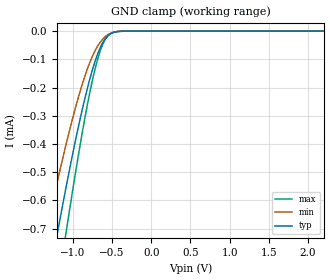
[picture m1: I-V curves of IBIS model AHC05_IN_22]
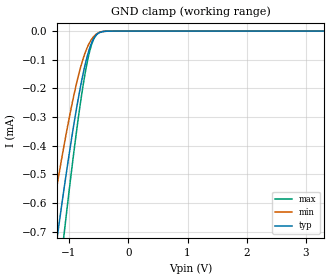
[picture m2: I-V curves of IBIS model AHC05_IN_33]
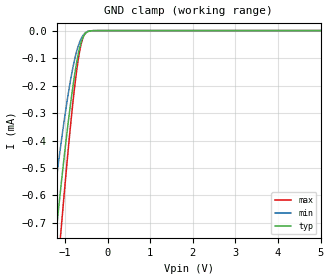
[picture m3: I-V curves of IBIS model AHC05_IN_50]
| TEXAS INSTRUMENTS INCORPORATED
| Standard Linear and Logic Group
| IBIS Model of SN74AHC05
| HEX INVERTERS WITH OPEN-DRAIN OUTPUTS
| This file contains package information for the following:
|  TSSOP 14-pin (PW) package as [Component] AHC05_PD_PW
|  PDIP 14-pin (N) package as [Component] AHC05_PD_N
|  SSOP 14-pin (DB) package as [Component] AHC05_PD_DB
|  SOIC 14-pin (D) package as [Component] AHC05_PD_D
|  TVSOP 14-pin (DGV) package as [Component] AHC05_PD_DGV
| This device can be powered at the following Vccs:
|  2.2 volt Vcc
|  3.3 volt Vcc
|  5 volt Vcc
| This file provides unique models under the [Model Selector] for each Vcc.
| For operation at a specific Vcc, select the appropriate model after each
| [Model Selector] keyword.
[IBIS Ver]   3.2
[Comment char]  |_char
[File Name]   sn74ahc05.ibs
[File Rev]   1.1 | i_die
[Date]   August 22, 2002
[Source]   Data created from TI-SPICE simulations at TI-SLL.
[Notes]   The following is an IBIS list for the AHC05_PD.
   Please contact sllibis@ti.com with questions and
   comments concerning SLL IBIS models.
[Disclaimer] Property of Texas Instruments Incorporated.  Unauthorized
   reproduction and/or distribution is strictly prohibited.
   This product is protected under copyright law.
   Created  2002, (C) Copyright  2002, Texas Instruments
   Incorporated, All Rights Reserved
   UNLESS THERE IS A SIGNED, WRITTEN AGREEMENT TO THE
   CONTRARY, TEXAS INSTRUMENTS (TI) IS PROVIDING THE IBIS
   MODELS  AND WITHOUT ANY WARRANTY, EXPRESSED OR
   IMPLIED.  TI assumes no liability for:
   1) the accuracy of the IBIS models provided to your
   company;
   2) the proper functioning of these IBIS Models in your
   design or for any resulting applications; or
   3) infringement of patents, copyrights or intellectual
   property rights resulting from your use of these IBIS
   models.
   TI provides IBIS Models as a service to our customers.
   You and your company shall not distribute, sell or give
   these models to anyone else without prior written
   permission from TI.
   TI reserves the right to make changes to our products or
   to discontinue any semiconductor product or service
   without notice, and advises our customers to obtain the
   latest version of relevant information to verify, before
   placing orders, that the information being relied on is
   current.
   Please be aware that your receipt and use of the IBIS
   information provided shall serve as acceptance of these
   terms and conditions.  If you do not accept these terms,
   you should return or destroy the IBIS models and any
   other accompanying information immediately.
| Component AHC05_PD_PW 14-pin TSSOP
[Component]   AHC05_PW
[Manufacturer]   Texas Instruments, Inc.
[Package]
|   typ   min   max
R_pkg   3.200e-02   2.900e-02   3.500e-02
L_pkg   2.378e-09   2.170e-09   2.680e-09
C_pkg   3.140e-13   2.700e-13   3.350e-13
[Pin]   signal_name   model_name   R_pin   L_pin   C_pin
1   1A   AHC05_IN   3.300e-02   2.618e-09   3.300e-13
2   1Y   AHC05_OUT   3.100e-02   2.313e-09   3.170e-13
3   2A   AHC05_IN   3.000e-02   2.310e-09   3.140e-13
4   2Y   AHC05_OUT   3.100e-02   2.173e-09   2.720e-13
5   3A   AHC05_IN   3.000e-02   2.204e-09   3.090e-13
6   3Y   AHC05_OUT   3.200e-02   2.315e-09   3.170e-13
7   GND   GND   3.500e-02   2.680e-09   3.350e-13
8   4Y   AHC05_OUT   3.300e-02   2.640e-09   3.330e-13
9   4A   AHC05_IN   3.400e-02   2.347e-09   3.190e-13
10   5Y   AHC05_OUT   2.900e-02   2.277e-09   3.130e-13
11   5A   AHC05_IN   3.100e-02   2.170e-09   2.700e-13
12   6Y   AHC05_OUT   3.100e-02   2.244e-09   3.110e-13
13   6A   AHC05_IN   3.300e-02   2.343e-09   3.210e-13
14   VCC   POWER   3.500e-02   2.657e-09   3.320e-13
| Component AHC05_PD_N 14-pin PDIP
[Component]   AHC05_N
[Manufacturer]   Texas Instruments, Inc.
[Package]
|   typ   min   max
R_pkg   4.500e-02   3.700e-02   6.300e-02
L_pkg   5.407e-09   3.922e-09   6.942e-09
C_pkg   3.890e-13   2.050e-13   6.040e-13
[Pin]   signal_name   model_name   R_pin   L_pin   C_pin
1   1A   AHC05_IN   6.300e-02   6.942e-09   6.040e-13
2   1Y   AHC05_OUT   3.700e-02   6.200e-09   4.060e-13
3   2A   AHC05_IN   4.200e-02   4.389e-09   3.220e-13
4   2Y   AHC05_OUT   3.800e-02   3.922e-09   2.050e-13
5   3A   AHC05_IN   3.900e-02   4.301e-09   2.980e-13
6   3Y   AHC05_OUT   3.800e-02   5.329e-09   3.560e-13
7   GND   GND   5.300e-02   6.510e-09   5.440e-13
8   4Y   AHC05_OUT   5.300e-02   6.437e-09   5.390e-13
9   4A   AHC05_IN   3.900e-02   5.352e-09   3.470e-13
10   5Y   AHC05_OUT   4.200e-02   4.473e-09   2.970e-13
11   5A   AHC05_IN   4.400e-02   4.326e-09   2.250e-13
12   6Y   AHC05_OUT   4.200e-02   4.295e-09   2.800e-13
13   6A   AHC05_IN   4.200e-02   6.318e-09   4.180e-13
14   VCC   POWER   6.100e-02   6.900e-09   6.030e-13
| Component AHC05_PD_DB 14-pin SSOP
[Component]   AHC05_DB
[Manufacturer]   Texas Instruments, Inc.
[Package]
|   typ   min   max
R_pkg   4.400e-02   4.100e-02   4.600e-02
L_pkg   3.551e-09   3.258e-09   3.927e-09
C_pkg   4.020e-13   3.600e-13   4.210e-13
[Pin]   signal_name   model_name   R_pin   L_pin   C_pin
1   1A   AHC05_IN   4.600e-02   3.927e-09   4.080e-13
2   1Y   AHC05_OUT   4.400e-02   3.587e-09   4.210e-13
3   2A   AHC05_IN   4.100e-02   3.289e-09   3.980e-13
4   2Y   AHC05_OUT   4.200e-02   3.258e-09   3.600e-13
5   3A   AHC05_IN   4.100e-02   3.286e-09   4.030e-13
6   3Y   AHC05_OUT   4.400e-02   3.586e-09   4.210e-13
7   GND   GND   4.600e-02   3.927e-09   4.080e-13
8   4Y   AHC05_OUT   4.600e-02   3.927e-09   4.080e-13
9   4A   AHC05_IN   4.400e-02   3.586e-09   4.210e-13
10   5Y   AHC05_OUT   4.100e-02   3.286e-09   4.030e-13
11   5A   AHC05_IN   4.300e-02   3.258e-09   3.600e-13
12   6Y   AHC05_OUT   4.100e-02   3.289e-09   3.980e-13
13   6A   AHC05_IN   4.400e-02   3.587e-09   4.210e-13
14   VCC   POWER   4.600e-02   3.927e-09   4.080e-13
| Component AHC05_PD_D 14-pin SOIC
[Component]   AHC05_D
[Manufacturer]   Texas Instruments, Inc.
[Package]
|   typ   min   max
R_pkg   3.100e-02   2.800e-02   3.400e-02
L_pkg   3.109e-09   2.462e-09   3.889e-09
C_pkg   4.730e-13   3.630e-13   6.280e-13
[Pin]   signal_name   model_name   R_pin   L_pin   C_pin
1   1A   AHC05_IN   3.300e-02   3.854e-09   6.220e-13
2   1Y   AHC05_OUT   3.200e-02   3.188e-09   4.730e-13
3   2A   AHC05_IN   2.800e-02   2.462e-09   3.770e-13
4   2Y   AHC05_OUT   3.100e-02   2.596e-09   3.630e-13
5   3A   AHC05_IN   2.800e-02   2.521e-09   3.720e-13
6   3Y   AHC05_OUT   3.400e-02   3.250e-09   4.760e-13
7   GND   GND   3.400e-02   3.889e-09   6.280e-13
8   4Y   AHC05_OUT   3.400e-02   3.889e-09   6.280e-13
9   4A   AHC05_IN   3.400e-02   3.250e-09   4.760e-13
10   5Y   AHC05_OUT   2.800e-02   2.521e-09   3.720e-13
11   5A   AHC05_IN   3.100e-02   2.596e-09   3.640e-13
12   6Y   AHC05_OUT   2.800e-02   2.462e-09   3.770e-13
13   6A   AHC05_IN   3.200e-02   3.188e-09   4.730e-13
14   VCC   POWER   3.300e-02   3.854e-09   6.220e-13
| Component AHC05_PD_DGV 14-pin TVSOP
[Component]   AHC05_DGV
[Manufacturer]   Texas Instruments, Inc.
[Package]
|   typ   min   max
R_pkg   3.500e-02   2.000e-02   4.500e-02
L_pkg   2.499e-09   2.077e-09   2.966e-09
C_pkg   3.610e-13   3.050e-13   4.160e-13
[Pin]   signal_name   model_name   R_pin   L_pin   C_pin
1   1A   AHC05_IN   2.700e-02   2.717e-09   3.730e-13
2   1Y   AHC05_OUT   3.700e-02   2.434e-09   3.980e-13
3   2A   AHC05_IN   3.400e-02   2.200e-09   3.160e-13
4   2Y   AHC05_OUT   2.000e-02   2.077e-09   3.090e-13
5   3A   AHC05_IN   3.000e-02   2.147e-09   3.050e-13
6   3Y   AHC05_OUT   4.200e-02   2.580e-09   4.080e-13
7   GND   GND   3.900e-02   2.921e-09   3.850e-13
8   4Y   AHC05_OUT   3.300e-02   2.841e-09   3.800e-13
9   4A   AHC05_IN   4.200e-02   2.611e-09   4.100e-13
10   5Y   AHC05_OUT   3.800e-02   2.331e-09   3.290e-13
11   5A   AHC05_IN   2.600e-02   2.223e-09   3.190e-13
12   6Y   AHC05_OUT   3.400e-02   2.259e-09   3.130e-13
13   6A   AHC05_IN   4.500e-02   2.681e-09   4.160e-13
14   VCC   POWER   4.200e-02   2.966e-09   3.860e-13
| Model AHC05_IN
[Model Selector]   AHC05_IN
AHC05_IN_22   2.2 volt Vcc
AHC05_IN_33   3.3 volt Vcc
AHC05_IN_50   5 volt Vcc
| Model AHC05_OUT
[Model Selector]   AHC05_OUT
AHC05_OUT_22   2.2 volt Vcc
AHC05_OUT_33   3.3 volt Vcc
AHC05_OUT_50   5 volt Vcc
| Models and submodels in the file (6): AHC05_IN_22 (Input), AHC05_IN_33 (Input), AHC05_IN_50 (Input), AHC05_OUT_22 (Open_drain), AHC05_OUT_33 (Open_drain), AHC05_OUT_50 (Open_drain)
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[Model]   AHC05_IN_22
Model_type  Input
Vinl = 0.5
Vinh = 1.5
| variable   typ   min   max
C_comp   0.89pF   0.81pF   0.98pF
[Temperature Range]   40   100   -40
| Ambient temperature   25   85   -40
[Voltage range]   2.2   2   2.4
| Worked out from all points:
|   GND clamp passes 1 mA (typ) near -1.38 V on its own axis
[GND Clamp]
| AHC05_IN_22
|   Voltage   I(typ)   I(min)   I(max)
-5.5V     -8.851mA   -7.354mA   -10.02mA
-1.355V   -959.3uA   -729.8uA   -1.218mA
-1.305V   -880.8uA   -665.9uA   -1.122mA
-1.205V   -727.2uA   -541.3uA   -931.7uA
-1.16V    -659.9uA   -487uA     -847.7uA
-1.09V    -557.7uA   -405.2uA   -719.4uA
-1.07V    -529.2uA   -382.5uA   -683.3uA
-895mV    -295.8uA   -201.7uA   -383.4uA
-745mV    -132.1uA   -85.68uA   -167uA
-635mV    -49.36uA   -33.72uA   -57.78uA
-530mV    -11.54uA   -9.155uA   -11.04uA
2.2V      580.3pA    219.9pA    1.028nA
[Model]   AHC05_IN_33
Model_type  Input
Vinl = 0.9
Vinh = 2.1
| variable   typ   min   max
C_comp   0.89pF   0.78pF   1.00pF
[Temperature Range]   40   100   -40
| Ambient temperature   25   85   -40
[Voltage range]   3.3   3   3.6
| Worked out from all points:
|   GND clamp passes 1 mA (typ) near -1.38 V on its own axis
[GND Clamp]
| AHC05_IN_33
|   Voltage   I(typ)   I(min)   I(max)
-5.5V     -8.851mA   -7.354mA   -10.02mA
-1.375V   -991uA     -755.7uA   -1.257mA
-1.32V    -904.2uA   -685uA     -1.15mA
-1.175V   -682.2uA   -505uA     -875.6uA
-1.085V   -550.6uA   -399.5uA   -710.3uA
-1.065V   -522.1uA   -376.9uA   -674.3uA
-895mV    -295.8uA   -201.7uA   -383.4uA
-800mV    -186.7uA   -122.7uA   -239.7uA
-730mV    -118.5uA   -76.84uA   -149uA
-620mV    -41.44uA   -28.88uA   -47.61uA
-505mV    -7.613uA   -6.114uA   -6.771uA
3.3V      1.837nA    303.9pA    8.84nA
[Model]   AHC05_IN_50
Model_type  Input
Vinl = 1.65
Vinh = 3.85
| variable   typ   min   max
C_comp   0.88pF   0.77pF   1.00pF
[Temperature Range]   40   100   -40
| Ambient temperature   25   85   -40
[Voltage range]   5   4.5   5.5
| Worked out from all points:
|   GND clamp passes 1 mA (typ) near -1.38 V on its own axis
[GND Clamp]
| AHC05_IN_50
|   Voltage   I(typ)   I(min)   I(max)
-5.5V     -8.851mA   -7.354mA   -10.02mA
-1.37V    -983.1uA   -749.2uA   -1.247mA
-1.315V   -896.4uA   -678.6uA   -1.141mA
-1.21V    -734.8uA   -547.4uA   -941.1uA
-1.11V    -586.6uA   -428.2uA   -755.8uA
-1.085V   -550.6uA   -399.5uA   -710.3uA
-905mV    -308.2uA   -210.9uA   -399.5uA
-810mV    -197.4uA   -130.2uA   -253.9uA
-730mV    -118.5uA   -76.84uA   -149uA
-610mV    -36.66uA   -25.92uA   -41.55uA
-480mV    -4.927uA   -3.935uA   -4.07uA
5V        7.166nA    474.1pA    66.12nA
